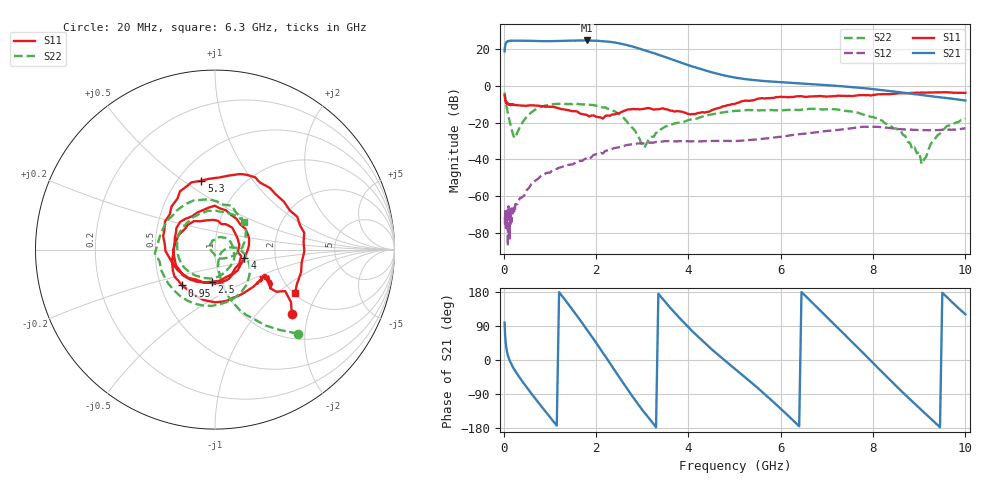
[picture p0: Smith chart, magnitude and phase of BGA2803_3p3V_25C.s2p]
#  HZ  S  RI  R  50.0000
! Rohde & Schwarz ZVA/B
! Temperature 25C
! Device number 102
! Measured Vcc 3.300000
! Measured Icc 0.006700
! DeltaGain  -0.177239  3dBBWHighMHz 2797.74  3dBBWLowMHz 29.77
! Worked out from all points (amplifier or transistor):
!   242 points, 20 MHz to 10 GHz, reference 50 ohm
!   highest |S21| = 24.7 dB at 1.8 GHz (marker M1)
!   |S21| within 3 dB of that: 31.93 MHz to 2.741 GHz (2.709 GHz wide, 195 % of centre)
!   unconditionally stable (mu >= 1): start of sweep to end of sweep
!   at 220 MHz: K = 58.40, MAG = 25.0 dB, |S12| = -66.8 dB
!   at 4 GHz: K = 4.32, MAG = 11.5 dB, |S12| = -30.3 dB
!   at 10 GHz: K = 10.42, MAG = -5.6 dB, |S12| = -23.1 dB
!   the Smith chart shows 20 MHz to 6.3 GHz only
!   S11 on the Smith chart (normalised r, x): 20 MHz: 1.52, -1.57; 950 MHz: 0.64, -0.28; 2.5 GHz: 0.90, -0.34; 4 GHz: 1.38, -0.13; 5.3 GHz: 0.65, +0.59; 6.3 GHz: 2.03, -1.33
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2e7  0.4278 -0.3571  -1.3 8.61  0.000186 0.000183  0.4618 -0.4685
3.5e7  0.3415 -0.2346  6.819 11.08  0.000339 0.000242  0.2239 -0.3907
6e7  0.2862 -0.163  13.59 7.892  -0.000125 6.54e-05  0.0809 -0.2717
1.6e8  0.2645 -0.1629  16.73 -2.931  -0.000139 -0.000432  0.0178 -0.0727
3.5e8  0.1849 -0.2254  11.6 -12.48  -0.000819 -0.000265  0.0736 0.0116
5.5e8  0.064 -0.2861  2.799 -16.67  -0.00145 0.00081  0.164 -0.0237
9.5e8  -0.1838 -0.1996  -13.13 -10.06  0.000781 0.00423  0.0738 -0.2885
1.3e9  -0.2271 0.02  -16.14 4.809  0.00529 0.00361  -0.229 -0.2265
1.7e9  -0.0489 0.1627  -2.253 17.09  0.00889 -0.00121  -0.2908 0.1143
1.8e9  0.0168 0.1605  2.808 17.04  0.0101 -0.0035  -0.2325 0.1932
2.2e9  0.1461 -0.0364  16.12 2.908  0.0092 -0.0141  0.0935 0.2448
2.5e9  -0.0188 -0.1793  10.2 -10.17  -0.00373 -0.0208  0.164 0.0424
2.7e9  -0.1796 -0.1424  2.128 -12.44  -0.0147 -0.02  0.0864 -0.0401
2.95e9  -0.2257 0.0336  -5.643 -8.55  -0.0254 -0.00925  0.000951 -0.0343
3.35e9  -0.0636 0.2214  -7.019 0.6266  -0.0264 0.0136  -0.0046 0.0533
4e9  0.1641 -0.0473  0.221 3.667  0.00748 0.0297  0.1091 -0.0418
5.05e9  -0.2419 0.2407  1.464 -0.7615  0.0274 -0.0155  -0.2072 -0.0248
5.3e9  -0.0755 0.3839  0.8981 -1.186  0.0207 -0.026  -0.2037 0.0827
6.3e9  0.4458 -0.2431  -1.142 -0.3468  -0.0387 -0.0257  0.1602 0.1552
6.7e9  0.0889 -0.5072  -0.9564 0.5551  -0.0523 0.00669  0.2348 0.00826
8.35e9  0.206 0.5561  0.4669 -0.5595  0.0691 -0.0181  -0.0685 -0.039
1e10  -0.0815 -0.6403  -0.2023 0.3428  -0.0663 -0.0214  -0.1256 -0.0246
